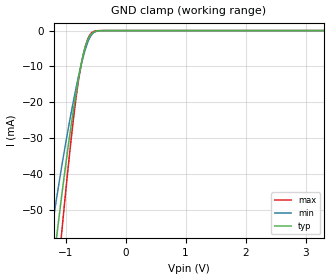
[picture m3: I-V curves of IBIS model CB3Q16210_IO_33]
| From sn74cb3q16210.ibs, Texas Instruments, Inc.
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[Model]   CB3Q16210_IO_33
Model_type  Terminator
| variable   typ   min   max
C_comp   3.28pF   2.67pF   3.97pF
| C_tri-state   3.28pF   2.67pF   3.97pF
[Temperature Range]   40   100   -40
| Ambient temperature   25   85   -40
[Voltage range]   3.3   3   3.6
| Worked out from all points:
|   GND clamp passes 1 mA (typ) near -0.57 V on its own axis
[GND Clamp]
| CB3Q16210_IO_33
|   Voltage   I(typ)   I(min)   I(max)
-5.5V     -867.9mA   -713.7mA   -1.031A
-1.245V   -71.43mA   -57.29mA   -89.68mA
-1.22V    -67.79mA   -54.51mA   -84.93mA
-1.15V    -57.82mA   -46.91mA   -71.88mA
-1.125V   -54.36mA   -44.26mA   -67.32mA
-1.065V   -46.24mA   -38.08mA   -56.59mA
-895mV    -25.12mA   -21.93mA   -28.61mA
-785mV    -13.46mA   -12.86mA   -14.03mA
-670mV    -4.456mA   -5.245mA   -4.445mA
-550mV    -651.5uA   -848.1uA   -420.8uA
-325mV    -1.904uA   -3.571uA   -165.1nA
3.3V      145.2pA    572.4pA    35.62pA
